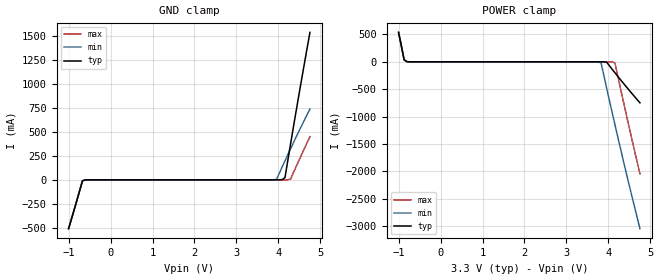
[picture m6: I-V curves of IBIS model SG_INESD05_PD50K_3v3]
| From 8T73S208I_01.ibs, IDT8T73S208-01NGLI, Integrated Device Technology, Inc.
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[Model] SG_INESD05_PD50K_3v3
Model_type   Input
Polarity   Non-Inverting
Vinl = 0.8V
Vinh = 2.0V
|   typ   min   max
C_comp   2pF   1.5pF   2.5pF
|   typ   min   max
[Voltage range]   3.3V   3.135V   3.465V
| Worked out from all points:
|   GND clamp passes 1 mA (typ) near -0.58 V on its own axis
|   POWER clamp passes 1 mA (typ) near -0.75 V on its own axis
[GND_clamp]
|Voltage   I (typ)   I (min)   I (max)
-999mV    -508.2mA   -508.2mA   -508.2mA
-668.6mV  -9.923mA   -9.923mA   -9.923mA
-602.5mV  -1.426mA   -1.426mA   -1.426mA
3.891V    87.97uA    775uA      77.07uA
3.957V    132.3uA    6.85mA     79.02uA
4.089V    2.173mA    134.9mA    105.8uA
4.155V    23.03mA    198mA      199.9uA
4.287V    371mA      322.2mA    6.957mA
4.486V    879.9mA    504mA      200.4mA
4.75V     1.535A     737.9mA    449.5mA
[Power_clamp]
|Voltage   I (typ)   I (min)   I (max)
-999mV    537.1mA    537.1mA    537.1mA
-866.8mV  35.03mA    35.03mA    35.04mA
-800.8mV  3.222mA    3.219mA    3.225mA
3.627V    -7.574uA   -146.9uA   -3.2uA
3.759V    -70.73uA   -2.461mA   -6.164uA
3.825V    -291uA     -21.02mA   -10.49uA
3.957V    -6.731mA   -479.5mA   -148.2uA
4.089V    -136.7mA   -928.9mA   -2.488mA
4.155V    -200.6mA   -1.15A     -21.32mA
4.42V     -450.3mA   -2.014A    -943.4mA
4.75V     -748.5mA   -3.045A    -2.045A
